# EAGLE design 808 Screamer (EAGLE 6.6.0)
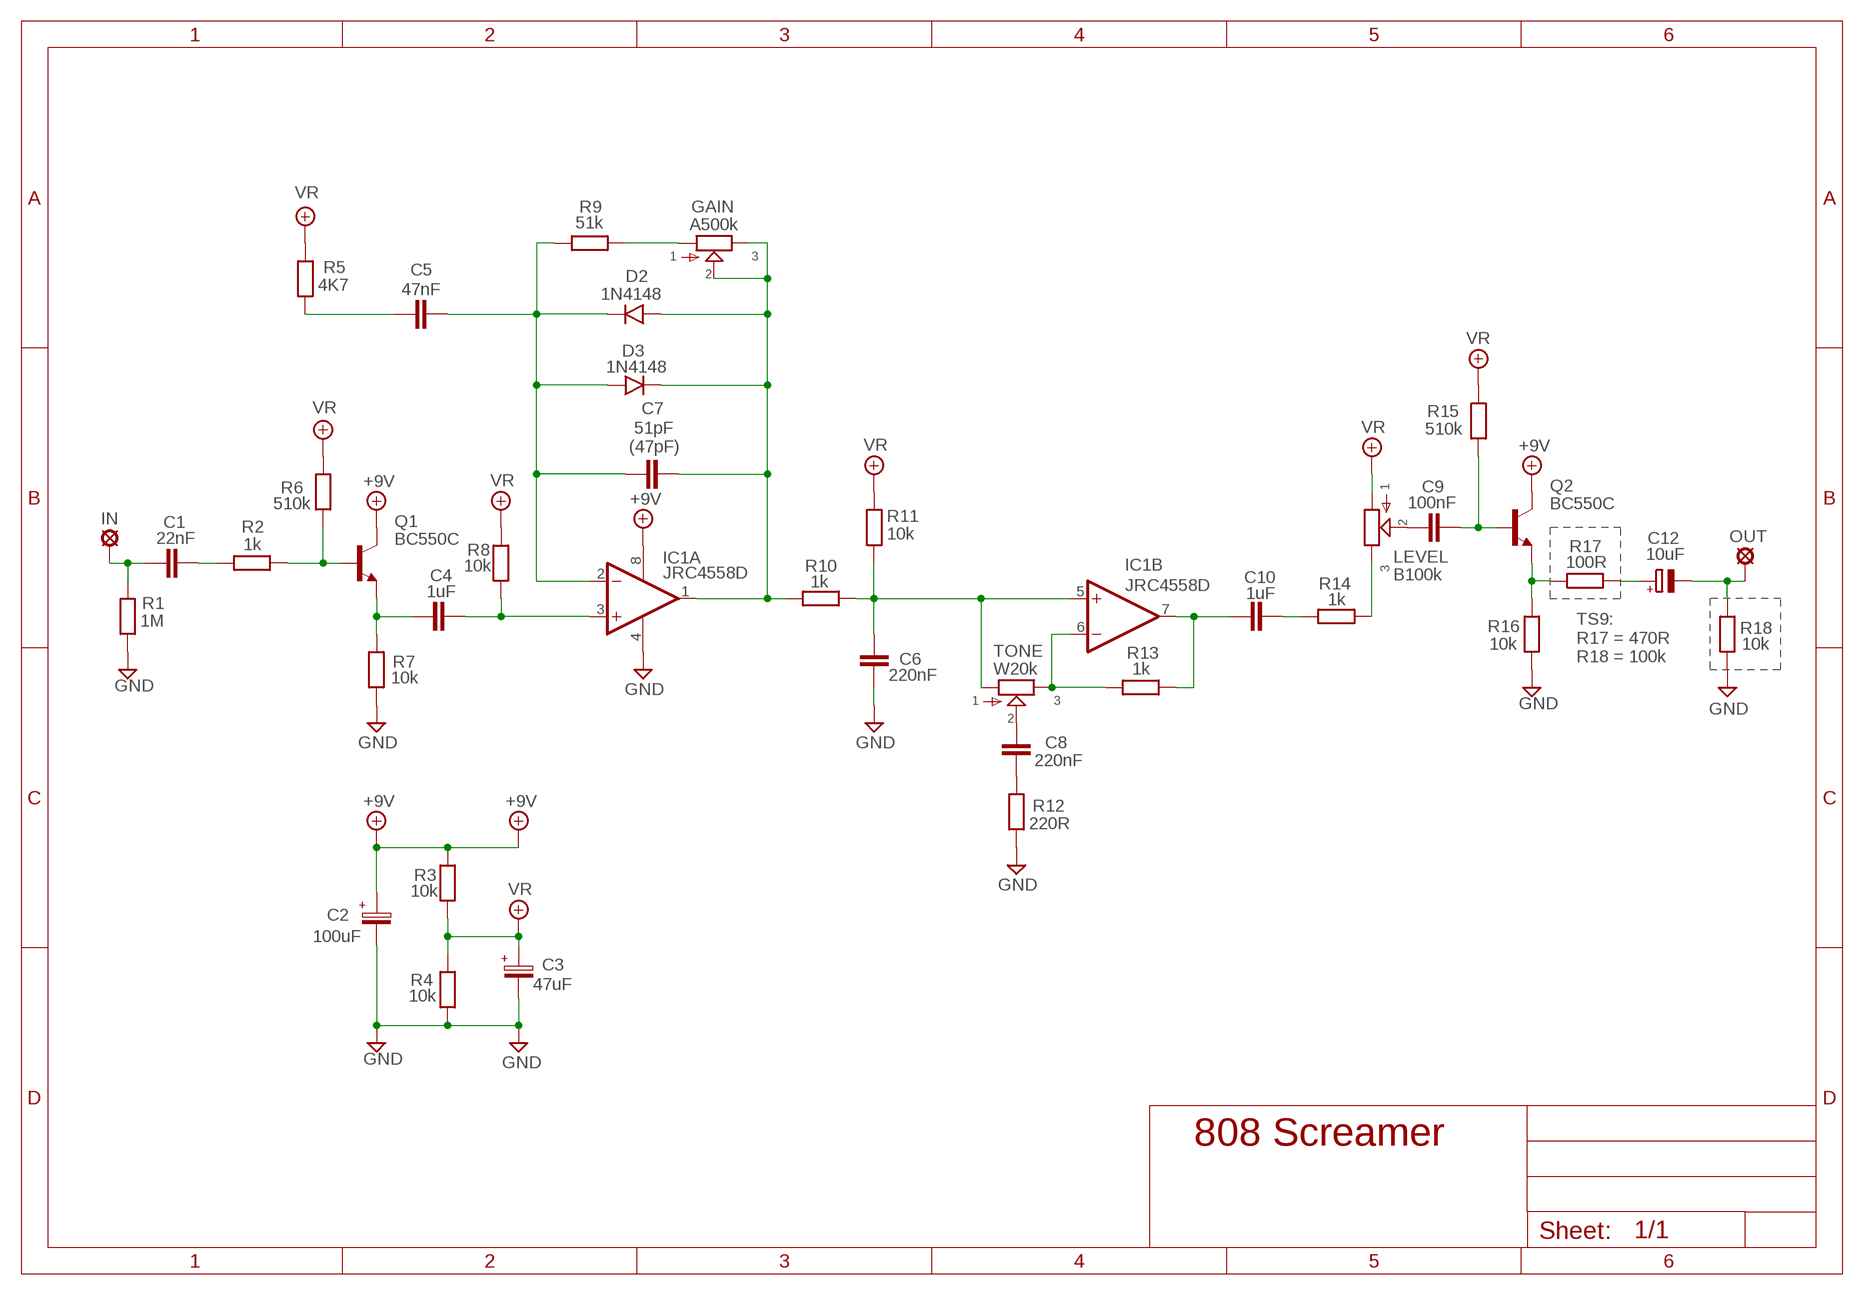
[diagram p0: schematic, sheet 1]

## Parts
+9V  +9V  +9V(T)1  [ROUND]
C1  22nF  072X0252  [072X025]
C2  100uF  063-EU  [063_025]
C3  47uF  063-EU  [063_025]
C4  1uF  072X0352  [072X035]
C5  47nF  072X0252  [072X025]
C6  220nF  072X0352  [072X035]
C7  51pF  050X030_0251  [050X030_025]
C8  220nF  072X0352  [072X035]
C9  100nF  072X0252  [072X025]
C10  1uF  072X0352  [072X035]
C12  10uF  CPOL-EUE5-4  [E5-4]
D2  1N4148  1N4148-3  [DO35-3]
D3  1N4148  1N4148-3  [DO35-3]
GAIN  A500k  POT-EU16MM  [16MM]
GND  GND  GND(T)1  [ROUND]
GND1  GND  GND(T)1  [ROUND]
IC1  JRC4558D  LM4558N  [DIL08]
IN  MCS10B  [MCS10B]
LEVEL  B100k  POT-EU16MM  [16MM]
OUT  MCS10B  [MCS10B]
Q1  BC550C  [TO92-EBC]
Q2  BC550C  [TO92-EBC]
R1  1M  6MM-EU3  [R0207/3]
R2  1k  6MM-EU3  [R0207/3]
R3  10k  6MM-EU3  [R0207/3]
R4  10k  6MM-EU3  [R0207/3]
R5  4K7  6MM-EU3  [R0207/3]
R6  510k  6MM-EU3  [R0207/3]
R7  10k  6MM-EU3  [R0207/3]
R8  10k  6MM-EU3  [R0207/3]
R9  51k  6MM-EU3  [R0207/3]
R10  1k  6MM-EU3  [R0207/3]
R11  10k  6MM-EU3  [R0207/3]
R12  220R  6MM-EU3  [R0207/3]
R13  1k  6MM-EU3  [R0207/3]
R14  1k  6MM-EU3  [R0207/3]
R15  510k  6MM-EU3  [R0207/3]
R16  10k  6MM-EU3  [R0207/3]
R17  100R  6MM-EU3  [R0207/3]
R18  10k  6MM-EU3  [R0207/3]
TONE  W20k  POT-EU16MM  [16MM]

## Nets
+9V: +9V.1(+9V) C2.+ IC1.8(P:V+) Q1.C Q2.C R3.2
GND: C2.- C3.- C6.2 GND1.1(GND) GND.1(GND) IC1.4(P:V-) R1.1 R4.1 R7.1 R12.1 R16.1 R18.1
N$1: C8.1 TONE.2
N$2: C1.2 R2.1
N$3: Q1.B R2.2 R6.1
N$4: C4.2 IC1.3(A:+IN) R8.1
N$5: C5.2 C7.1 D2.C D3.A IC1.2(A:-IN) R9.1
N$6: C4.1 Q1.E R7.2
N$7: C8.2 R12.2
N$8: GAIN.1 R9.2
N$9: C9.1 LEVEL.2
N$10: IC1.6(B:-IN) R13.1 TONE.3
N$11: C6.1 IC1.5(B:+IN) R10.2 R11.1 TONE.1
N$14: C10.1 IC1.7(B:OUT) R13.2
N$15: C10.2 R14.1
N$16: LEVEL.3 R14.2
N$17: Q2.E R16.2 R17.1
N$18: C1.1 IN.MP R1.2
N$19: C9.2 Q2.B R15.1
N$20: C12.+ R17.2
N$21: C12.- OUT.MP R18.2
N$22: C7.2 D2.A D3.C GAIN.2 GAIN.3 IC1.1(A:OUT) R10.1
N$23: C5.1 R5.1
VR: C3.+ LEVEL.1 R3.1 R4.2 R5.2 R6.2 R8.2 R11.2 R15.2

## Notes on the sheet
- (47pF)
- TS9:
  R17 = 470R
  R18 = 100k

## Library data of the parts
+9V = gm-supply:+9V(T): +9V Voltage Supply
C1 C5 C9 = Wima MKS:072X025: 1000pF - 0.47uF
C2 C3 = Elektrolyytit:063-EU
C4 C6 C8 C10 = Wima MKS:072X035: 0.15 - 1.0uF;
C7 = Keraamiset kondensaattorit:050X030_025: 47 - 120pF
C12 = rcl:CPOL-EU: POLARIZED CAPACITOR, European symbol
D2 D3 = Diodit:1N4148: Fast Switching Diode
GAIN LEVEL TONE = gm-pots:POT-EU
GND GND1 = gm-supply:GND(T): Ground
IC1 = Operaatiovahvistimet:*4558: *4558 Op Amp Infamous for its use in tube screamers. This op amp has many manufacturers, hence the leading "*" in the name. The JRC4558 is a widely used example.
IN OUT = Padit:MCS10B: SOLDER PAD
Q1 Q2 = transistor-npn:BC550*: NPN Transistor
R1-R18 = Vastukset:6MM-EU: 6mm Resistors (European schematic symbol)

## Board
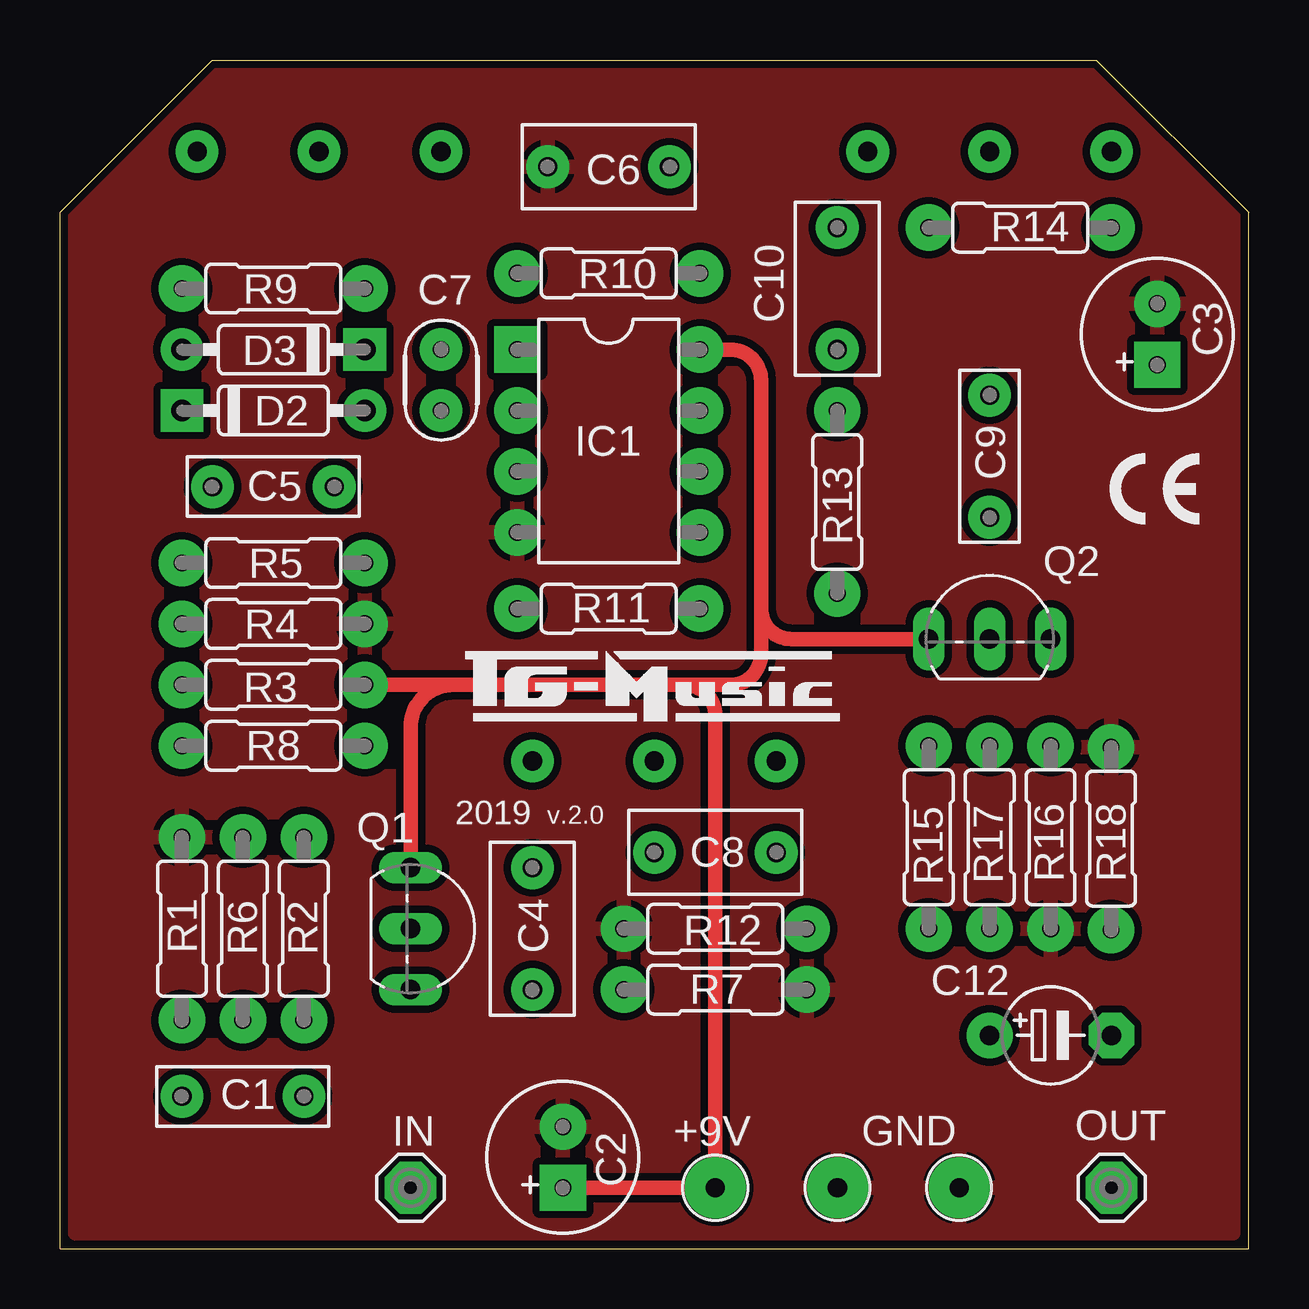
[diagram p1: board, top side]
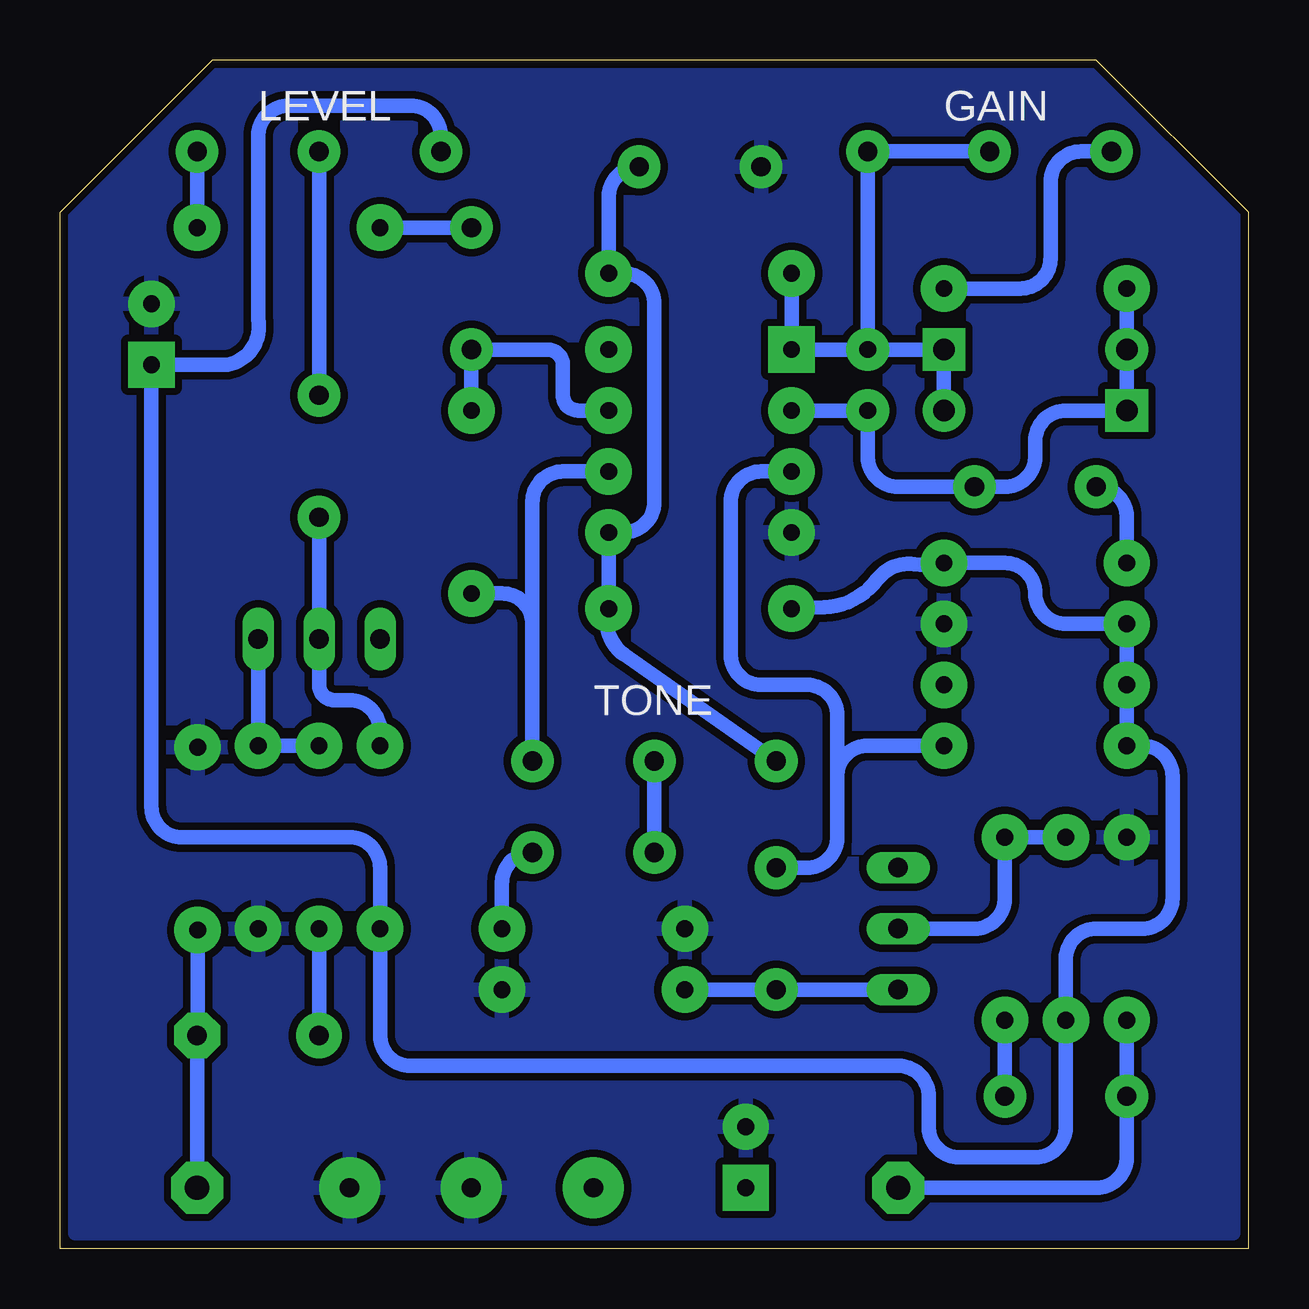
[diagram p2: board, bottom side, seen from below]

Size 49.53 x 49.53 mm. Coordinates in mm from the lower left corner, seen from the top.
Outline: 0,0 49.53,0 49.53,43.18 43.18,49.53 6.35,49.53 0,43.18 0,0
Copper layers (1*16): Top 0.035mm / dielectric 1.5mm / Bottom 0.035mm
Design rules "ITEADstudio": minimum track width 10mil, minimum drill 12mil, track to track 12mil, track to pad 12mil, pad to pad 12mil, via to via 12mil, smd to smd 0mil, copper to edge 12mil, drill to drill 12mil, minimum pad ring 10mil, minimum via ring 6mil, stop-mask expansion 4mil, vias tented up to drill 100mil, thermal gap 10mil

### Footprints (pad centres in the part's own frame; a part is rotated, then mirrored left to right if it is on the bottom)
ROUND = drill 0.8 pad 2.54: 1 0,0
072X025 = drill 0.8 pad 1.778: 1 -2.54,0; 2 2.54,0
063_025 = drill 0.7 pad 1.93 square: + -1.27,0 | drill 0.7 pad 1.93: - 1.27,0
072X035 = drill 0.8 pad 1.778: 1 -2.54,0; 2 2.54,0
050X030_025 = drill 0.7 pad 1.778: 1 -1.27,0; 2 1.27,0
E5-4 = drill 0.813 pad 1.905: + -2.54,0 | drill 0.813 pad 1.905 octagon: - 2.54,0
DO35-3 = drill 0.9 pad 1.778: A 3.81,0 | drill 0.9 pad 1.778 square: C -3.81,0
16MM = drill 0.8 pad 1.778: 1 5.08,0; 2 0,0; 3 -5.08,0
DIL08 = drill 0.7 pad 1.93 square: 1 -3.81,-3.81 | drill 0.7 pad 1.93: 2 -1.27,-3.81; 3 1.27,-3.81; 4 3.81,-3.81; 5 3.81,3.81; 6 1.27,3.81; 7 -1.27,3.81; 8 -3.81,3.81
MCS10B = drill 1.016 pad 2.159 octagon: MP 0,0
TO92-EBC = drill 0.813 long: B 0,-1.27; C -2.54,-1.27; E 2.54,-1.27
R0207/3 = drill 0.7 pad 1.93: 1 -3.81,0; 2 3.81,0

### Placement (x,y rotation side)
+9V  27.3,2.54 0 top
C1  7.62,6.35 0 top
C2  20.95,3.81 90 top
C3  45.72,38.1 90 top
C4  19.68,13.34 90 top
C5  8.89,31.75 0 top
C6  22.86,45.09 180 top
C7  15.88,36.2 90 top
C8  27.3,16.51 0 top
C9  38.73,33.02 270 top
C10  32.38,40.01 90 top
C12  41.27,8.89 0 top
D2  8.89,34.92 0 top
D3  8.89,37.47 180 top
GAIN  10.79,45.72 0 bottom
GND  32.4,2.54 0 top
GND1  37.47,2.54 0 top
IC1  22.86,33.66 270 top
IN  14.61,2.54 0 top
LEVEL  38.73,45.72 0 bottom
OUT  43.81,2.54 0 top
Q1  15.88,13.34 270 top
Q2  38.73,26.67 0 top
R1  5.08,13.34 270 top
R2  10.16,13.34 90 top
R3  8.89,23.5 0 top
R4  8.89,26.04 180 top
R5  8.89,28.57 0 top
R6  7.62,13.34 270 top
R7  27.3,10.79 180 top
R8  8.89,20.95 180 top
R9  8.89,40.01 0 top
R10  22.86,40.64 0 top
R11  22.86,26.67 180 top
R12  27.3,13.34 0 top
R13  32.38,31.11 90 top
R14  40.01,42.55 0 top
R15  36.2,17.14 270 top
R16  41.27,17.14 90 top
R17  38.73,17.14 270 top
R18  43.79,17.09 270 top
TONE  24.77,20.32 0 bottom

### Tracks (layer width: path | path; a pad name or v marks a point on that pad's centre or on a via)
+9V
  Top 0.61: C2.+ +9V.1 27.3,22.23 arc90 26.04,23.5 | R3.2 16.51,23.5 | 16.51,23.5 26.04,23.5 | 26.04,23.5 27.94,23.5 arc90 29.21,24.77 29.21,26.67 | 29.21,26.67 29.21,36.2 arc90 27.94,37.47 IC1.8 | Q2.C 30.48,25.4 arc-90 29.21,26.67 | Q1.C 14.61,21.72 arc-90 16.38,23.5 16.51,23.5
GND
  pour Bottom: 0.64,48.9 48.9,48.9 48.9,0.64 0.64,0.64
  pour Top: 0.64,0.64 0.64,43.18 6.35,48.9 43.18,48.9 48.9,43.18 48.9,0.64
N$1
  Bottom 0.61: TONE.2 C8.1
N$2
  Bottom 0.61: C1.2 R2.1
N$3
  Bottom 0.61: R6.1 R2.2 10.16,14.61 arc90 11.43,13.34 Q1.B
N$4
  Bottom 0.61: R8.1 15.88,20.95 arc-90 17.14,19.68 | 17.14,19.68 17.14,17.14 arc90 18.41,15.88 C4.2 | IC1.3 20.32,32.38 arc-90 21.59,31.11 21.59,24.77 arc-90 20.32,23.5 18.41,23.5 arc90 17.14,22.23 17.14,19.68
N$5
  Bottom 0.61: R9.1 D3.A D2.C 7.62,34.92 arc-90 8.89,33.66 8.89,33.02 arc90 10.16,31.75 C5.2 14.61,31.75 arc90 15.88,33.02 C7.1 IC1.2
N$6
  Bottom 0.61: Q1.E C4.1 R7.2
N$7
  Bottom 0.61: R12.2 31.11,15.24 arc90 C8.2
N$8
  Bottom 0.61: GAIN.1 6.99,45.72 arc-90 8.26,44.45 8.26,41.27 arc90 9.53,40.01 R9.2
N$9
  Bottom 0.61: LEVEL.2 C9.1
N$10
  Bottom 0.61: R13.1 31.11,27.3 arc90 29.84,26.04 | 29.84,26.04 TONE.3 | IC1.6 28.57,32.38 arc-90 29.84,31.11 29.84,26.04
N$11
  Bottom 0.61: TONE.1 26.04,24.77 arc73 R11.1 IC1.5 26.04,29.84 arc-90 24.77,31.11 24.77,39.37 arc-90 26.04,40.64 R10.2 26.67,43.81 arc90 C6.1
N$14
  Bottom 0.61: R13.2 C10.1 29.21,37.47 arc90 28.57,36.83 28.57,35.56 arc-90 27.94,34.92 IC1.7
N$15
  Bottom 0.61: C10.2 R14.1
N$16
  Bottom 0.61: LEVEL.3 R14.2
N$17
  Bottom 0.61: R17.1 R16.2 Q2.E
N$18
  Bottom 0.61: IN.MP 6.35,2.54 arc-90 5.08,3.81 C1.1 R1.2
N$19
  Bottom 0.61: C9.2 Q2.B 38.73,23.5 arc-90 38.1,22.86 37.47,22.86 arc90 36.2,21.59 R15.1
N$20
  Bottom 0.61: C12.+ R17.2
N$21
  Bottom 0.61: R18.2 43.79,9.55 arc90 C12.- OUT.MP
N$22
  Bottom 0.61: GAIN.2 GAIN.3 C7.2 | R10.1 IC1.1 C7.2 | D2.A D3.C C7.2
N$23
  Bottom 0.61: R5.1 5.08,30.48 arc-90 C5.1
VR
  Bottom 0.61: R11.2 17.69,26.72 arc-51 15.49,27.87 arc60 13.94,28.52 arc-20 R5.2 10.16,28.57 arc90 8.89,27.3 arc-90 7.62,26.04 R4.2 R3.1 R8.2 4.45,20.95 arc90 3.17,19.68 3.17,14.61 arc90 4.45,13.34 6.35,13.34 arc-90 7.62,12.06 R6.2 7.62,5.08 arc90 8.89,3.81 12.06,3.81 arc90 13.34,5.08 13.34,6.35 arc-90 14.61,7.62 34.92,7.62 arc90 36.2,8.89 R15.2 36.2,15.88 arc-90 37.47,17.14 44.45,17.14 arc90 45.72,18.41 C3.+ 42.55,36.83 arc-90 41.27,38.73 41.27,46.35 arc90 40.01,47.62 34.92,47.62 arc90 33.66,46.35 LEVEL.1

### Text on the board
tNames: 2019 | v.2.0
